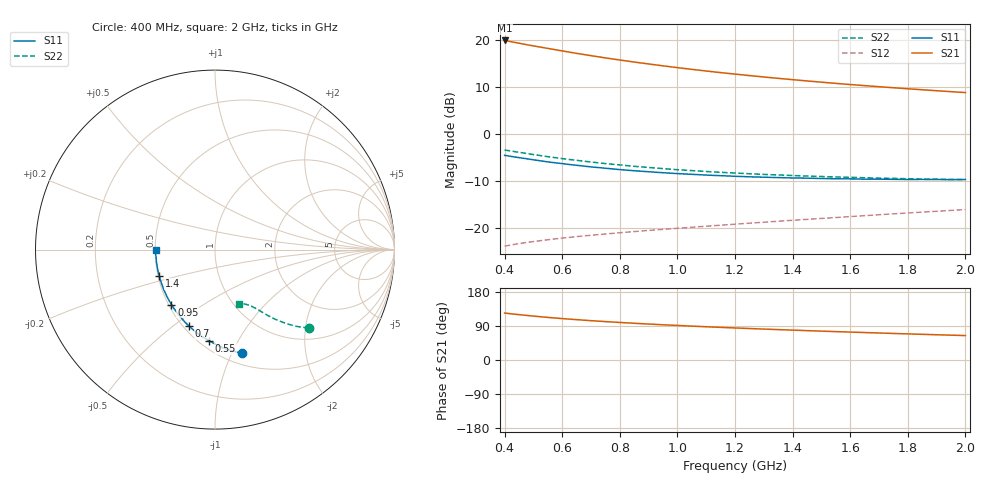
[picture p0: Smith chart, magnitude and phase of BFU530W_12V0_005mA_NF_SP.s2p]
! Filename:  P:\Prog\Test\Noise\ATS_data\Testdata_Net\06 Compressed Noise after Statistics\BFU530W_APM2013_09_A05_12p0V_005mA_NF_CM01_D.sf
! Date/Time: Tue 26/Mar/2013 18:06:02
! BFU530W_APM2013_09_A05_12p0V_1to25mA_NF_CM01_Bias4_R.sf
! Noise Parameter Data File
! BFU530W_APM2013_09_A05_12p0V_1to25mA_NF_CM01
! Date/time: Thu Mar 21 22:54:15 2013
! VAR V_out= 12.000000
! VAR I_out= 4.990000
! VAR V_in= 0.800900
! VAR I_in= 0.041905
! Device data file deembeded for feedlines and parallel
! Original file: \06 Compressed Noise after Statistics\BFU530W_APM2013_09_A05_12p0V_005mA_NF_CM01_R.sf
! Feed-files: PR019V01_070313_Feed1.s2p, PR019V01_070313_Feed2.s2p
! Parallel-file: PR019V01_070313_Par.s2p
# MHz S MA R 50
!  Freq-MHz  S11-mag  S11-arg  S21-mag  S21-arg  S12-mag  S12-arg  S22-mag  S22-arg
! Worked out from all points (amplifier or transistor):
!   37 points, 400 MHz to 2 GHz, reference 50 ohm
!   highest |S21| = 19.9 dB at 400 MHz (marker M1)
!   |S21| within 3 dB of that: start of sweep to 676.9 MHz
!   unconditionally stable (mu >= 1): 1.801 GHz to end of sweep
!   at 500 MHz: K = 0.50, MSG = 20.8 dB, |S12| = -22.8 dB
!   at 1.1 GHz: K = 0.84, MSG = 16.5 dB, |S12| = -19.5 dB
!   at 2 GHz: K = 1.01, MAG = 11.7 dB, |S12| = -16.0 dB
!   lowest NFmin = 0.62 dB at 420 MHz
!   S11 on the Smith chart (normalised r, x): 400 MHz: 0.61, -1.10; 550 MHz: 0.56, -0.77; 700 MHz: 0.53, -0.57; 950 MHz: 0.52, -0.37; 1.4 GHz: 0.51, -0.17; 2 GHz: 0.50, -0.00
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400  0.5971 -75.4  9.888 123.9  0.06488 56.7  0.6802 -39.8
420  0.5832 -78.1  9.627 122.1  0.06665 56.1  0.665 -40.8
440  0.5705 -80.7  9.374 120.5  0.06825 55.5  0.65 -41.7
480  0.5472 -85.7  8.881 117.4  0.07124 54.5  0.6224 -43.4
500  0.5354 -88.2  8.657 115.9  0.07262 54.1  0.6087 -44.1
550  0.5087 -93.7  8.144 112.4  0.07589 53.4  0.5782 -45.7
600  0.4876 -99.1  7.661 109.2  0.07904 52.8  0.551 -47.1
650  0.468 -103.9  7.213 106.5  0.08195 52.4  0.5285 -48.3
700  0.4501 -108.7  6.822 103.8  0.08466 52.2  0.5072 -49.5
750  0.4358 -113.0  6.457 101.4  0.08736 52.1  0.4881 -50.3
800  0.4214 -117.2  6.133 99.1  0.09009 52.1  0.4723 -51.2
850  0.4098 -121.2  5.837 96.9  0.09267 52.2  0.4567 -51.9
950  0.3903 -128.4  5.319 93.0  0.09785 52.5  0.4317 -53.3
1050  0.3755 -135.1  4.881 89.4  0.103 53.0  0.411 -54.5
1100  0.3687 -138.2  4.688 87.7  0.1057 53.3  0.4023 -55.1
1200  0.358 -144.2  4.347 84.6  0.111 53.9  0.3876 -56.2
1300  0.35 -149.7  4.051 81.6  0.1165 54.5  0.3746 -57.2
1400  0.3436 -154.8  3.793 78.8  0.1221 55.0  0.3644 -58.4
1500  0.339 -159.5  3.568 76.2  0.1278 55.5  0.356 -59.6
1650  0.3336 -166.2  3.279 72.5  0.1367 56.2  0.3453 -61.4
1750  0.3322 -170.2  3.115 70.1  0.1429 56.6  0.34 -62.6
2000  0.3311 -179.7  2.769 64.5  0.1587 57.3  0.3299 -66.1
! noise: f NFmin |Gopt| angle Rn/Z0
400  0.6486  0.1637  33.06  0.1142
460  0.6661  0.1613  38.68  0.1096
600  0.6749  0.1805  47.3  0.115
800  0.6927  0.1885  62.4  0.1117
1000  0.7571  0.2002  75.84  0.1036
1200  0.8025  0.2041  92.08  0.0981
1400  0.8107  0.2076  111.4  0.0923
1600  0.8274  0.2293  120.5  0.0788
1800  0.8698  0.2357  139  0.0748
2000  0.8808  0.2731  150.2  0.069
